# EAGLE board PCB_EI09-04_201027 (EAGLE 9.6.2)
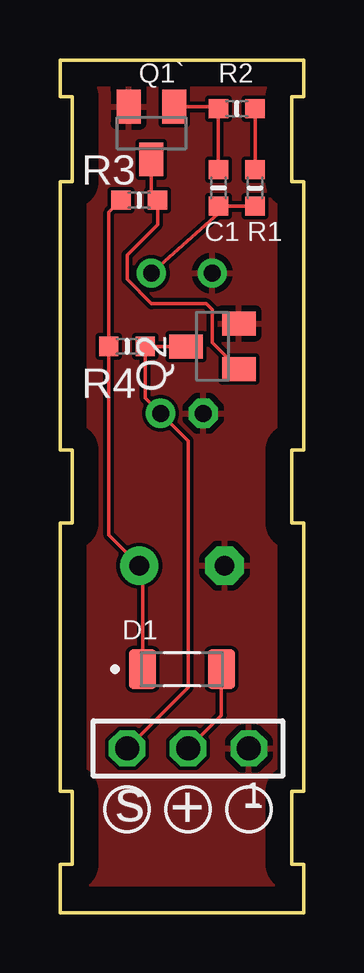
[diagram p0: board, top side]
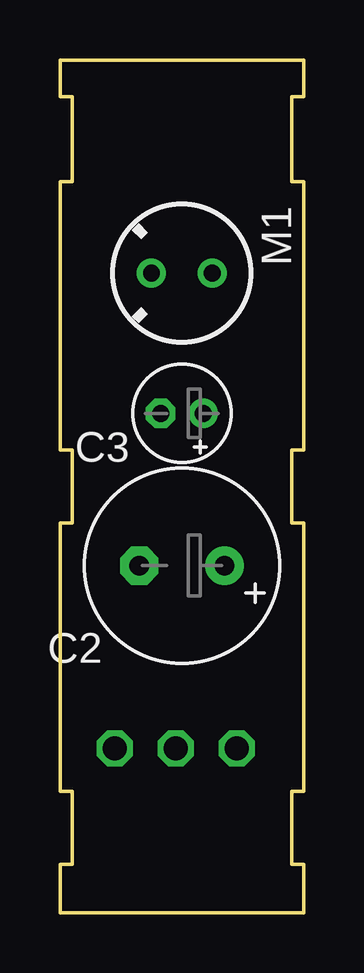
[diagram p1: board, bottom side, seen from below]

Size 10.16 x 35.56 mm. Coordinates in mm from the lower left corner, seen from the top.
Outline: 0,0 10.16,0 10.16,2.03 9.65,2.03 9.65,5.08 10.16,5.08 10.16,16.26 9.65,16.26 9.65,19.3 10.16,19.3 10.16,30.48 9.65,30.48 9.65,34.04 10.16,34.04 10.16,35.56 0,35.56 0,34.04 0.51,34.04 0.51,30.48 0,30.48 0,19.3 0.51,19.3 0.51,16.26 0,16.26 0,5.08 0.51,5.08 0.51,2.03 0,2.03 0,0
Copper layers (1*16): Top 0.035mm / dielectric 1.5mm / Bottom 0.035mm
Design rules "default": minimum track width 6mil, minimum drill 0.35mm, track to track 6mil, track to pad 6mil, pad to pad 6mil, via to via 6mil, smd to smd 6mil, copper to edge 40mil, drill to drill 6mil, minimum pad ring 10mil, minimum via ring 8mil, stop-mask expansion 4mil, vias tented up to drill 0mil, thermal gap 10mil

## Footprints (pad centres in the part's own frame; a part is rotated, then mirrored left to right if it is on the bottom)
RC-MASTER-SMD_C0603MP = smd 0.8 x 0.8: 1 -0.762,0; 2 0.762,0
E3,5-8 = drill 0.813 pad 1.6: + -1.778,0 | drill 0.813 pad 1.6 octagon: - 1.778,0
E1,8-4 = drill 0.711 pad 1.168: + -0.889,0 | drill 0.711 pad 1.168 octagon: - 0.889,0
DIOMELF3414N = smd 1.14 x 1.63: A 1.64,0; C -1.64,0
F6050AP = drill 0.7 pad 1.2: 1 0,1.27; 2 0,-1.27
SOT23-BEC = smd 1 x 1.4: B -0.95,-1.1; C 0,1.1; E 0.95,-1.1
RC-MASTER-SMD_R0603MP = smd 0.8 x 0.8: 1 -0.762,0; 2 0.762,0
TSW-103-XX-G-S = drill 1 pad 1.5 octagon: 1 2.54,0; 2 0,0; 3 -2.54,0

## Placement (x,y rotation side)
C1  1uF  [RC-MASTER-SMD_C0603MP]  6.6,30.23 270 top
C2  470uF  [E3,5-8]  5.08,14.48 180 bottom
C3  100uF  [E1,8-4]  5.08,20.83 180 bottom
D1  FDLL4148  [DIOMELF3414N]  5.08,10.16 0 top
M1  ELECTRET_MICROPHON-F6050AP  [F6050AP]  5.08,26.67 270 bottom
Q1`  MMBT2222ALT1  [SOT23-BEC]  3.81,32.51 180 top
Q2  MMBT2222ALT1  [SOT23-BEC]  6.35,23.62 90 top
R1  2K  [RC-MASTER-SMD_R0603MP]  8.13,30.23 90 top
R2  910K  [RC-MASTER-SMD_R0603MP]  7.37,33.53 180 top
R3  10K  [RC-MASTER-SMD_R0603MP]  3.3,29.72 0 top
R4  4.7K  [RC-MASTER-SMD_R0603MP]  2.79,23.62 0 top
X1  TSW-103-07-G-S  [TSW-103-XX-G-S]  5.33,6.86 0 top

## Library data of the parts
C1 R1-R4 = 52101-101-REV-A_v16
C2 C3 = rcl; SPICEPREFIX: C
D1 = FDLL4148; DESCRIPTION: Diode Standard 100V 200mA Surface Mount SOD-80; DIGI-KEY_PART_NUMBER: FDLL4148CT-ND; MF: ON Semiconductor; MP: FDLL4148; PACKAGE: SOD-80-2 ON Semiconductor; PURCHASE-URL: https://pricing.snapeda.com/search/part/FDLL4148/?ref=eda
M1 = microphon
Q1` Q2 = transistor-neu-to92
X1 = con-samtec; MF: Samtec Inc.; MPN: TSW-103-07-G-S

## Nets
GND: C2.- C3.- M1.2 Q1`.E Q2.E X1.1
N$1: D1.A X1.2
N$2: C3.+ Q2.C R4.2 X1.3
N$3: C1.1 Q1`.B R2.2
N$4: R1.2 R2.1
N$5: C1.2 M1.1 R1.1
N$6: Q1`.C Q2.B R3.2
N$7: C2.+ D1.C R3.1 R4.1

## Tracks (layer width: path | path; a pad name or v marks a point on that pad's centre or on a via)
GND
  pour Top: 0,35.56 10.16,35.56 10.16,0 0,0
N$1
  Top 0.152: X1.2 6.72,8.24 D1.A
N$2
  Top 0.152: X1.3 5.33,9.4 5.33,19.68 C3.+ 3.56,21.46 R4.2 Q2.C
N$3
  Top 0.152: Q1`.B 6.52,33.61 R2.2 C1.1
N$4
  Top 0.152: R2.1 R1.2
N$5
  Top 0.152: R1.1 C1.2 6.6,29.14 M1.1
N$6
  Top 0.152: Q2.B 6.35,23.77 6.35,25.15 6.1,25.4 3.81,25.4 2.79,26.42 2.79,27.43 4.06,28.7 R3.2 3.81,29.97 Q1`.C
N$7
  Top 0.152: D1.C 3.44,14.34 C2.+ 2.03,15.75 R4.1 2.03,29.21 R3.1

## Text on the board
tPlace: s | + | -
